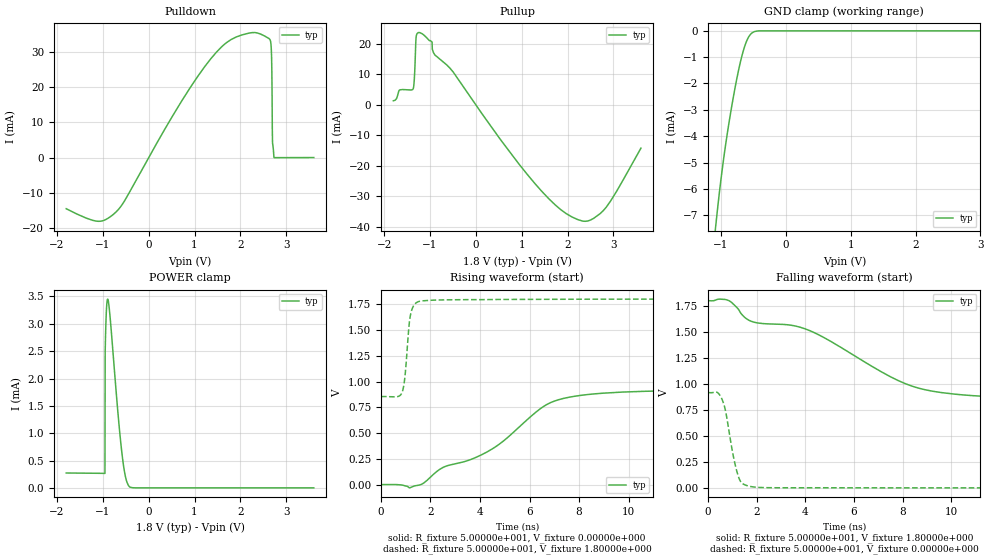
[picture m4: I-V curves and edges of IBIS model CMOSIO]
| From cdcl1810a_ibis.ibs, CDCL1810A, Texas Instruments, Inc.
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|   Model CMOSIO
[Model]   CMOSIO
Model_type   I/O
Vinl   = 6.00000e-001
Vinh   = 1.20000e+000
Vmeas  = 9.00000e-001
Cref   = 0.00000e+000
Rref   = 2.50000e+001
Vref   = 9.00000e-001
|   typ   min   max
C_comp   9.00000e-013   9.00000e-013   9.00000e-013
[Temperature Range]   2.70000e+001   NA   NA
|   |   typ   min   max
[Voltage Range]   1.80000e+000   NA   NA
[Pullup Reference]   1.80000e+000   NA   NA
[Pulldown Reference]   0.00000e+000   NA   NA
[POWER Clamp Reference]   1.80000e+000   NA   NA
[GND Clamp Reference]   0.00000e+000   NA   NA
[Ramp]
R_load = 5.000e+001
|   typ   min   max
dV/dt_r 5.494e-001/3.727e-009   NA   NA
dV/dt_f 5.677e-001/6.028e-009   NA   NA
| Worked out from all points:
|   slope of the pulldown table from 0 to 0.27 V, typ, clamps not added: 43 ohm
|   slope of the pullup table from 0 to 0.27 V, typ, clamps not added: 46.7 ohm
|   GND clamp passes 1 mA (typ) near -0.68 V on its own axis
|   POWER clamp passes 1 mA (typ) near -0.63 V on its own axis
|   rising waveform, R_fixture 5.00000e+001, V_fixture 0.00000e+000: 20-80 % time 3.73ns typ, NA min, NA max; typ from 0 V to 0.916 V
|   rising waveform, R_fixture 5.00000e+001, V_fixture 1.80000e+000: 20-80 % time 201ps typ, NA min, NA max; typ from 0.854 V to 1.8 V
|   falling waveform, R_fixture 5.00000e+001, V_fixture 1.80000e+000: 20-80 % time 6.03ns typ, NA min, NA max; typ from 1.8 V to 0.854 V
|   falling waveform, R_fixture 5.00000e+001, V_fixture 0.00000e+000: 20-80 % time 431ps typ, NA min, NA max; typ from 0.916 V to 0 V
[Pullup]
| Voltage   I(typ)   I(min)   I(max)
-1.8V     1.364mA    NA         NA
-1.665V   4.889mA    NA         NA
-1.365V   5.359mA    NA         NA
-1.34V    9.032mA    NA         NA
-1.3V     22.59mA    NA         NA
-1.175V   23.39mA    NA         NA
-955mV    20.62mA    NA         NA
1.28V     -25.65mA   NA         NA
1.85V     -34.33mA   NA         NA
2.325V    -38.1mA    NA         NA
2.835V    -33.7mA    NA         NA
3.6V      -14.18mA   NA         NA
[Pulldown]
| Voltage   I(typ)   I(min)   I(max)
-1.8V     -14.6mA    NA         NA
-1.11V    -18.17mA   NA         NA
-720mV    -15.6mA    NA         NA
1.21V     25.73mA    NA         NA
2.17V     35.44mA    NA         NA
2.655V    33.25mA    NA         NA
2.68V     28.25mA    NA         NA
2.685V    24.6mA     NA         NA
2.695V    8.297mA    NA         NA
2.7V      4.109mA    NA         NA
2.735V    -30.96uA   NA         NA
3.6V      0A         NA         NA
[GND Clamp]
| Voltage   I(typ)   I(min)   I(max)
-1.8V     -28.25mA   NA         NA
-1.08V    -7.362mA   NA         NA
-1V       -5.615mA   NA         NA
-925mV    -4.249mA   NA         NA
-850mV    -3.079mA   NA         NA
-760mV    -1.856mA   NA         NA
-690mV    -1.067mA   NA         NA
-620mV    -480.7uA   NA         NA
-555mV    -161.6uA   NA         NA
-495mV    -40.21uA   NA         NA
-410mV    -1.503uA   NA         NA
3.6V      0A         NA         NA
[POWER Clamp]
| Voltage   I(typ)   I(min)   I(max)
-1.8V     271.8uA    NA         NA
-955mV    264.1uA    NA         NA
-950mV    2.488mA    NA         NA
-940mV    2.846mA    NA         NA
-925mV    3.215mA    NA         NA
-895mV    3.452mA    NA         NA
-850mV    3.19mA     NA         NA
-675mV    1.406mA    NA         NA
-585mV    636uA      NA         NA
-505mV    195.2uA    NA         NA
-420mV    20.45uA    NA         NA
3.6V      0A         NA         NA
[Rising Waveform]
R_fixture   = 5.00000e+001
V_fixture   = 0.00000e+000
C_fixture   = 0.00000e+000
| Time   V(typ)   V(min)   V(max)
0s        760.5nV    NA         NA
1.15ns    -32.43mV   NA         NA
1.65ns    3.737mV    NA         NA
2.5ns     164.9mV    NA         NA
3.625ns   242.7mV    NA         NA
4.475ns   342.8mV    NA         NA
6.45ns    738.5mV    NA         NA
7.325ns   833mV      NA         NA
9.75ns    897.5mV    NA         NA
14.98ns   915.7mV    NA         NA
[Rising Waveform]
R_fixture   = 5.00000e+001
V_fixture   = 1.80000e+000
C_fixture   = 0.00000e+000
| Time   V(typ)   V(min)   V(max)
0s        853.9mV    NA         NA
675ps     853.7mV    NA         NA
850ps     892.1mV    NA         NA
925ps     966.4mV    NA         NA
975ps     1.061V     NA         NA
1.125ns   1.52V      NA         NA
1.2ns     1.655V     NA         NA
1.325ns   1.738V     NA         NA
1.55ns    1.778V     NA         NA
14.98ns   1.8V       NA         NA
[Falling Waveform]
R_fixture   = 5.00000e+001
V_fixture   = 1.80000e+000
C_fixture   = 0.00000e+000
| Time   V(typ)   V(min)   V(max)
0s        1.8V       NA         NA
850ps     1.801V     NA         NA
1.5ns     1.641V     NA         NA
1.85ns    1.596V     NA         NA
3.4ns     1.564V     NA         NA
4.175ns   1.512V     NA         NA
7.45ns    1.075V     NA         NA
8.675ns   958mV      NA         NA
10.87ns   886.9mV    NA         NA
14.98ns   853.9mV    NA         NA
[Falling Waveform]
R_fixture   = 5.00000e+001
V_fixture   = 0.00000e+000
C_fixture   = 0.00000e+000
| Time   V(typ)   V(min)   V(max)
0s        915.7mV    NA         NA
375ps     918.1mV    NA         NA
575ps     851mV      NA         NA
725ps     731.6mV    NA         NA
1.025ns   320.7mV    NA         NA
1.225ns   124.8mV    NA         NA
1.375ns   48.56mV    NA         NA
1.65ns    18.16mV    NA         NA
2.7ns     1.24mV     NA         NA
14.98ns   760.5nV    NA         NA
